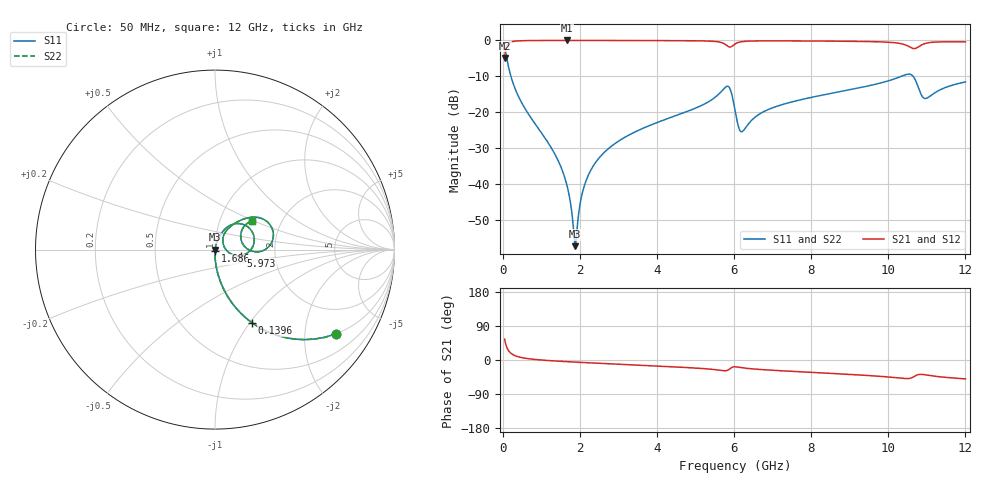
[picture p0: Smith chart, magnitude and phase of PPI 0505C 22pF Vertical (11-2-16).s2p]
# GHz S MA R 50
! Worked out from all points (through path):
!   1601 points, 50 MHz to 12 GHz, reference 50 ohm
!   highest |S21| = -0.01 dB at 1.671 GHz (marker M1); lowest = -4.9 dB at 50 MHz (marker M2)
!   group delay of S21, straight-line fit = 13.1 ps
!   lowest |S11| = -57.3 dB at 1.88 GHz (marker M3), VSWR 1.00, Z = 50.1 - j0.0218 ohm
!   |S11| at or under -10 dB: 213.5 MHz to 10.34 GHz (10.12 GHz wide, 192 % of centre); 10.64 GHz to end of sweep
!   |S22| runs from -57.3 to -1.7 dB; largest |S21 - S12| = 0
!   S11 on the Smith chart (normalised r, x): 50 MHz: 0.99, -2.87; 139.6 MHz: 0.99, -1.02; 1.686 GHz: 1.00, -0.02; 5.973 GHz: 1.34, -0.09; 12 GHz: 1.43, +0.50
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0.05  0.8216 -34.9  0.5699 55.1  0.5699 55.1  0.8216 -34.9
0.139625  0.4568 -63.2  0.8892 26.8  0.8892 26.8  0.4568 -63.2
0.259125  0.2634 -75.4  0.9641 14.5  0.9641 14.5  0.2634 -75.4
0.5354688  0.123 -84.2  0.9916 5.5  0.9916 5.5  0.123 -84.2
1.342094  0.02669 -90.0  0.9984 -2.5  0.9984 -2.5  0.02669 -90.0
1.670719  0.009383 -86.6  0.9986 -4.4  0.9986 -4.4  0.009383 -86.6
1.685656  0.008696 -86.0  0.9986 -4.5  0.9986 -4.5  0.008696 -86.0
1.879844  0.001357 -9.2  0.9985 -5.6  0.9985 -5.6  0.001357 -9.2
2.044156  0.006659 71.3  0.9984 -6.4  0.9984 -6.4  0.006659 71.3
2.268219  0.01493 76.7  0.9983 -7.6  0.9983 -7.6  0.01493 76.7
2.634187  0.02749 77.3  0.9978 -9.4  0.9978 -9.4  0.02749 77.3
4.038312  0.07288 72.0  0.9947 -16.1  0.9947 -16.1  0.07288 72.0
5.808406  0.2286 27.9  0.8535 -28.0  0.8535 -28.0  0.2286 27.9
5.972719  0.1494 -12.8  0.8509 -18.4  0.8509 -18.4  0.1494 -12.8
6.025  0.1069 -16.3  0.8928 -17.9  0.8928 -17.9  0.1069 -16.3
6.211719  0.05359 26.7  0.9624 -20.5  0.9624 -20.5  0.05359 26.7
6.809219  0.1042 59.3  0.9855 -25.9  0.9855 -25.9  0.1042 59.3
8.019156  0.1613 55.5  0.9813 -32.7  0.9813 -32.7  0.1613 55.5
10.01331  0.2742 41.3  0.9428 -44.9  0.9428 -44.9  0.2742 41.3
10.58094  0.3356 14.3  0.7975 -47.9  0.7975 -47.9  0.3356 14.3
10.96931  0.1552 19.5  0.9101 -39.3  0.9101 -39.3  0.1552 19.5
12  0.2639 37.8  0.9527 -49.8  0.9527 -49.8  0.2639 37.8
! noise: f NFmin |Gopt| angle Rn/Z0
0.05  0.0003932  0.8671  0.9993  0.0006358
1.372  0.004046  0.6781  4.181  0.002426
2.701  0.00677  0.6323  7.82  0.003445
4.031  0.009888  0.6268  11.44  0.004916
5.36  0.0248  0.784  15.54  0.02316
6.682  0.02623  0.7512  19.37  0.02067
8.012  0.02056  0.645  22.47  0.01057
9.341  0.02662  0.6767  26.11  0.01511
10.67  0.1647  0.9316  30.79  0.4978
12  0.03693  0.7011  33.47  0.02225
